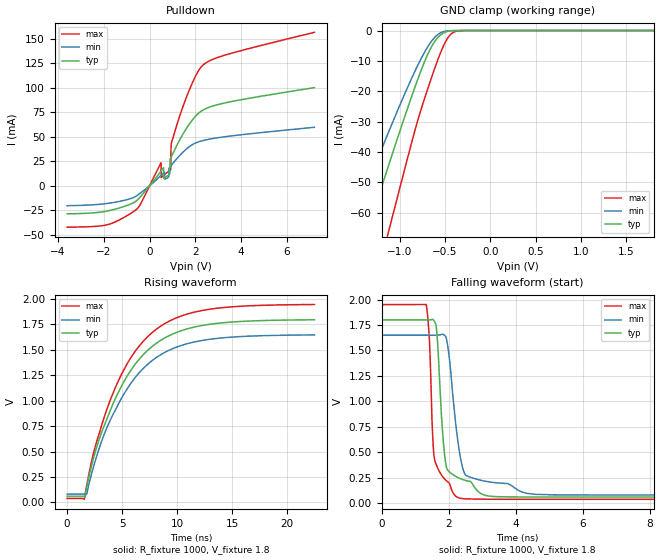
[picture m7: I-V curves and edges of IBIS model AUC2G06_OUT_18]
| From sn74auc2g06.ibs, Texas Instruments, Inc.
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[Model]   AUC2G06_OUT_18
Model_type  Open_drain
Enable   Active-Low
Vref =   0
Rref =   1000
Cref =   30p
Vmeas =   0.9
| variable   typ   min   max
C_comp   2.97pF   2.53pF   3.26pF
| C_pulldown   4.74pF   0.72pF   14.09pF
| C_tri-state   2.97pF   2.53pF   3.26pF
[Temperature Range]   40   100   -40
| Ambient temperature   25   85   -40
[Voltage range]   1.8   1.65   1.95
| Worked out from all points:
|   slope of the pulldown table from 0 to 0.27 V, typ, clamps not added: 34.3 ohm
|   GND clamp passes 1 mA (typ) near -0.53 V on its own axis
|   rising waveform, R_fixture 1000, V_fixture 1.8: 20-80 % time 4.56ns typ, 4.56ns min, 4.51ns max; typ from 0.061 V to 1.8 V
|   falling waveform, R_fixture 1000, V_fixture 1.8: 20-80 % time 213ps typ, 335ps min, 155ps max; typ from 1.8 V to 0.061 V
[GND Clamp]
| AUC2G06_OUT_18
|   Voltage   I(typ)   I(min)   I(max)
-3.6V     -279.3mA   -228.7mA   -348mA
-1.555V   -84.85mA   -65.88mA   -116.2mA
-1.365V   -66.96mA   -51.42mA   -94.33mA
-1.32V    -62.75mA   -48.04mA   -89.13mA
-1.125V   -44.68mA   -33.64mA   -66.54mA
-815mV    -17.24mA   -12.36mA   -31.12mA
-685mV    -7.459mA   -5.101mA   -18.71mA
-610mV    -3.475mA   -2.138mA   -12.15mA
-530mV    -1.024mA   -505.6uA   -5.921mA
-425mV    -87.51uA   -45.91uA   -946.5uA
-295mV    -1.872uA   -1.583uA   -13.35uA
1.8V      394.7pA    569.4pA    453.3pA
[Pulldown]
| AUC2G06_OUT_18
|   Voltage   I(typ)   I(min)   I(max)
-3.6V     -28.49mA   -20.22mA   -42.08mA
-690mV    -16.99mA   -11.76mA   -26.03mA
495mV     14.95mA    10.62mA    23.51mA
505mV     15.26mA    10.84mA    8.468mA
840mV     11.22mA    9.16mA     14.98mA
885mV     12.27mA    19.08mA    15.87mA
895mV     26.23mA    19.35mA    16.1mA
915mV     28.13mA    19.9mA     16.6mA
950mV     29.67mA    20.88mA    43.17mA
1.25V     43.93mA    29.26mA    66.37mA
2.385V    77.89mA    46.46mA    124mA
7.2V      100.1mA    59.68mA    156.4mA
[Ramp]
| AUC2G06_OUT_18
| variable   typ   min   max
dV/dt_r   1.05/4.56E-09   0.94/4.56E-09   1.15/4.51E-09
dV/dt_f   1.05/2.26E-10   0.95/3.44E-10   1.15/1.58E-10
R_load = 1000
[Rising Waveform]
| AUC2G06_OUT_18
R_fixture =   1000
C_fixture =   0
L_fixture =   0
V_fixture =   1.8
V_fixture_min = 1.65
V_fixture_max = 1.95
|   Time   V(typ)   V(min)   V(max)
0s        61.05mV    81.2mV     38.68mV
1.555ns   58.5mV     80.9mV     29.95mV
1.79ns    151.4mV    86.56mV    173.3mV
2.55ns    492.3mV    405.7mV    545.8mV
4.315ns   1.004V     892.7mV    1.11V
6.015ns   1.333V     1.204V     1.459V
7.995ns   1.555V     1.416V     1.693V
10.07ns   1.677V     1.532V     1.821V
12.74ns   1.748V     1.601V     1.896V
22.5ns    1.796V     1.647V     1.946V
[Falling Waveform]
| AUC2G06_OUT_18
R_fixture =   1000
C_fixture =   0
L_fixture =   0
V_fixture =   1.8
V_fixture_min = 1.65
V_fixture_max = 1.95
|   Time   V(typ)   V(min)   V(max)
0s        1.8V       1.65V      1.95V
1.33ns    1.8V       1.65V      1.951V
1.43ns    1.8V       1.65V      1.58V
1.575ns   1.786V     1.65V      439mV
1.655ns   1.646V     1.65V      359.1mV
1.91ns    399.1mV    1.637V     228.4mV
2.32ns    246.2mV    508.8mV    51.37mV
2.52ns    222.8mV    272mV      43.44mV
4.585ns   61.38mV    87.72mV    38.73mV
22.5ns    61.05mV    81.2mV     38.68mV
